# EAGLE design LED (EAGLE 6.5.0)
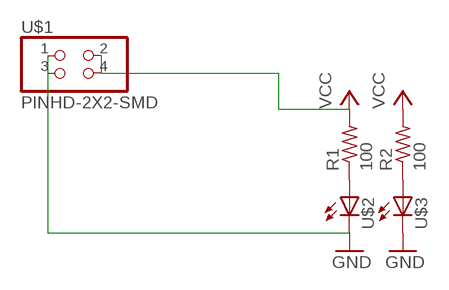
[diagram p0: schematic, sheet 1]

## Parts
R1  100  RES-US1206FAB  [R1206FAB]
R2  100  RES-US1206FAB  [R1206FAB]
U$1  PINHD-2X2-SMD  [2X02SMD]
U$2  LED1206  [1206]
U$3  LED1206  [1206]

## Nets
GND: U$1.1 U$1.3 U$2.2(C) U$3.2(C)
N$1: R1.1 U$2.1(A)
N$2: R2.1 U$3.1(A)
VCC: R1.2 R2.2 U$1.2 U$1.4

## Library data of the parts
R1 R2 = fab:RES-US: Resistor (US Symbol)
U$1 = fab:PINHD-2X2-SMD
U$2 U$3 = FabLab:LED

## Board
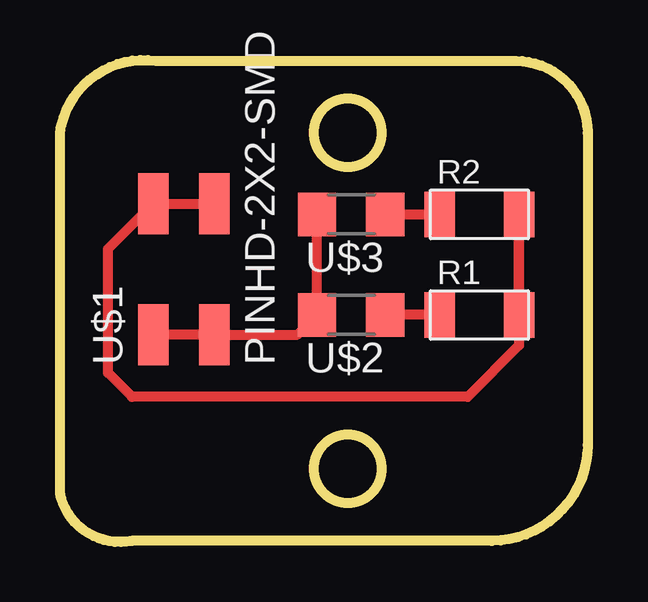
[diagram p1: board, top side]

Size 22 x 20.08 mm. Coordinates in mm from the lower left corner, seen from the top.
Outline: 4,20.05 19,20.05 arc-90 22,17.05 22,4.05 arc-90 18,0.05 3,0.05 arc-90 0,2.05 0,17.05 arc-90 4,20.05
Outline: circle at 12,3.05 radius 1.41
Outline: circle at 12,17.05 radius 1.41
Copper layers (1*16): Top 0.035mm / dielectric 1.5mm / Bottom 0.035mm
Design rules "default": minimum track width 10mil, minimum drill 24mil, track to track 8mil, track to pad 8mil, pad to pad 8mil, via to via 8mil, smd to smd 8mil, copper to edge 40mil, drill to drill 8mil, minimum pad ring 10mil, minimum via ring 8mil, stop-mask expansion 4mil, vias tented up to drill 0mil, thermal gap 10mil

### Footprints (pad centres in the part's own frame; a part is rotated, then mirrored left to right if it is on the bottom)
R1206FAB = smd 1.27 x 1.905: 1 -1.651,0; 2 1.651,0
2X02SMD = smd 2.54 x 1.27: 1 -2.54,1.27; 2 2.92,1.27; 3 -2.54,-1.27; 4 2.92,-1.27
1206 = smd 1.6 x 1.803: 1 -1.422,0; 2 1.422,0

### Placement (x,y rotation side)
R1  17.49,9.46 0 top
R2  17.49,13.65 0 top
U$1  5.16,11.18 90 top
U$2  12.14,9.46 180 top
U$3  12.14,13.65 180 top

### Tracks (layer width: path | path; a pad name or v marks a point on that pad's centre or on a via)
GND
  Top 0.406: U$1.1 U$1.3 9.9,8.64 U$2.2 U$3.2
N$1
  Top 0.406: R1.1 U$2.1
N$2
  Top 0.406: U$3.1 R2.1
VCC
  Top 0.406: U$1.4 U$1.2 2,12.21 2,7.05 3,6.05 17,6.05 19.14,8.19 R2.2 R1.2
